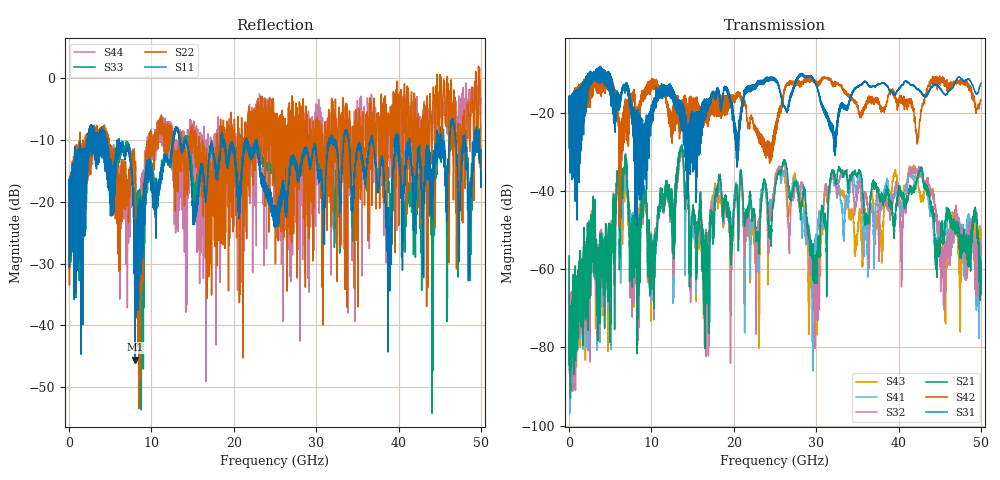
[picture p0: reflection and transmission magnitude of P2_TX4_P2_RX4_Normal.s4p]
!Keysight Technologies,N5225B,MY57041031,A.13.20.10
!Date: Friday, May 31, 2019 11:32:43
!Correction: S11(Full 4 Port(1,2,3,4))
!S12(Full 4 Port(1,2,3,4))
!S13(Full 4 Port(1,2,3,4))
!S14(Full 4 Port(1,2,3,4))
!S21(Full 4 Port(1,2,3,4))
!S22(Full 4 Port(1,2,3,4))
!S23(Full 4 Port(1,2,3,4))
!S24(Full 4 Port(1,2,3,4))
!S31(Full 4 Port(1,2,3,4))
!S32(Full 4 Port(1,2,3,4))
!S33(Full 4 Port(1,2,3,4))
!S34(Full 4 Port(1,2,3,4))
!S41(Full 4 Port(1,2,3,4))
!S42(Full 4 Port(1,2,3,4))
!S43(Full 4 Port(1,2,3,4))
!S44(Full 4 Port(1,2,3,4))
!S4P File: Measurements: <S11,S12,S13,S14>,
!<S21,S22,S23,S24>,
!<S31,S32,S33,S34>,
!<S41,S42,S43,S44>:
# Hz S  dB  R 50.0
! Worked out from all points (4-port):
!   5000 points, 10 MHz to 50 GHz, reference 50 ohm
!   strongest paths, dB at 10 MHz, 12.51 GHz, 25.01 GHz, 37.51 GHz, 50 GHz:
!     S31: -19.3, -14.3, -11.3, -12.8, -12.5
!     S42: -19.7, -27.8, -24.2, -17.2, -16.7
!     S21: -56.7, -45.9, -40.1, -39.5, -59.8
!     S32: -57.1, -47.4, -38.0, -44.3, -56.0
!     S41: -64.2, -48.1, -38.0, -40.6, -53.9
!     S43: -74.9, -48.8, -36.8, -48.1, -51.2
!   lowest |S11| = -45.5 dB at 8.03 GHz (marker M1), VSWR 1.01, Z = 50.2 - j0.487 ohm
!   |S11| at or under -10 dB: 6.073 GHz to 12.61 GHz (6.542 GHz wide, 70 % of centre); 14.21 GHz to 18.43 GHz (4.228 GHz wide, 25.9 % of centre); 22.71 GHz to 31.61 GHz (8.893 GHz wide, 32.7 % of centre)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
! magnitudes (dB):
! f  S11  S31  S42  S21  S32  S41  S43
! 10 MHz  -19.0  -19.3  -19.7  -56.7  -57.1  -64.2  -74.9
! 8.03 GHz  -45.5  -23.3  -16.8  -44.5  -47.7  -45.5  -49.4
! 25.98 GHz  -17.0  -18.0  -16.6  -32.8  -33.5  -35.1  -35.2
! 30.03 GHz  -12.1  -13.1  -11.9  -59.1  -62.1  -51.4  -62.0
! 31.91 GHz  -10.4  -24.9  -12.1  -35.1  -36.3  -35.9  -36.2
! 42.7 GHz  -13.9  -14.8  -20.1  -34.3  -35.6  -34.4  -42.4
! 50 GHz  -15.1  -12.5  -16.7  -59.8  -56.0  -53.9  -51.2
